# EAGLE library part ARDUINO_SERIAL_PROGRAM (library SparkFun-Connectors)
FTDI connector footprints
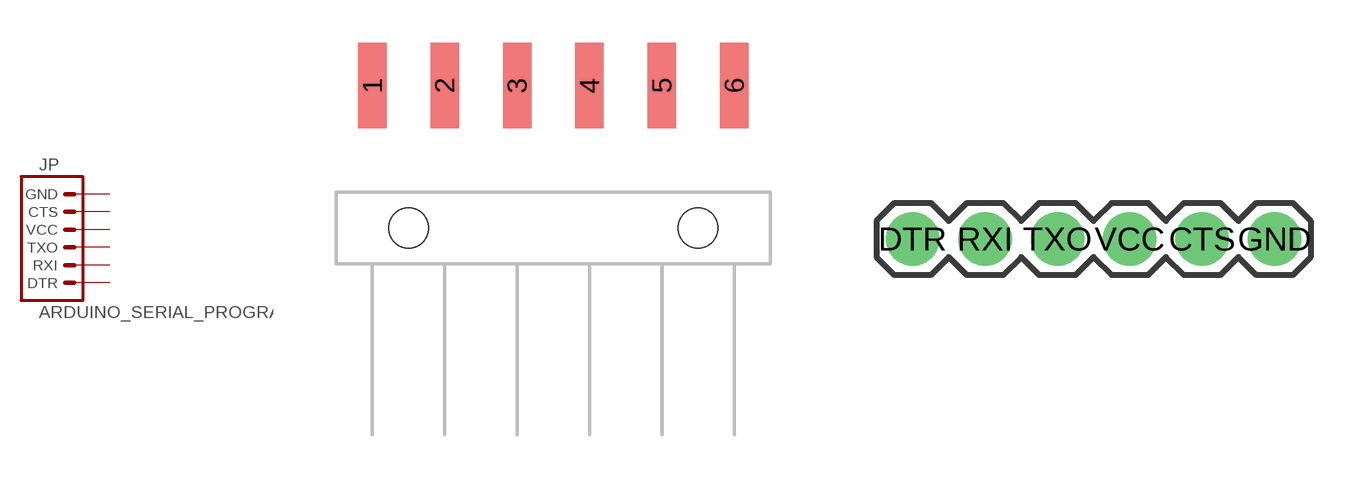
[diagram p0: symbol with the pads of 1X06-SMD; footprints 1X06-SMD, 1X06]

Designator prefix JP

## ARDUINO_SERIAL_PROGRAMSMD  [1X06-SMD]
1  DTR  pas
2  RXI  pas
3  TXO  pas
4  VCC  pas
5  CTS  pas
6  GND  pas

## ARDUINO_SERIAL_PROGRAMPTH  [1X06]
CTS  CTS  pas
DTR  DTR  pas
GND  GND  pas
RXI  RXI  pas
TXO  TXO  pas
VCC  VCC  pas

## ARDUINO_SERIAL_PROGRAMRA_LOCK  [MOLEX-1X6-RA_LOCK]
1  GND  pas
2  CTS  pas
3  VCC  pas
4  TXO  pas
5  RXI  pas
6  DTR  pas

## ARDUINO_SERIAL_PROGRAMLONGPADS  [1X06_LONGPADS]
Pads as for 1X06-SMD

## ARDUINO_SERIAL_PROGRAMLOCK  [1X06_LOCK]
Pads as for 1X06-SMD

## ARDUINO_SERIAL_PROGRAMPTH-KIT  [1X06-KIT]
Pads as for 1X06-SMD

## Footprint 1X06-SMD (pad centres in mm)
smd 1 x 3: 1 -6.35,5; 2 -3.81,5; 3 -1.27,5; 4 1.27,5; 5 3.81,5; 6 6.35,5
hole 1.4 at -5.08,0
hole 1.4 at 5.08,0

## Footprint 1X06 (pad centres in mm)
drill 1.016 pad 1.88: CTS 10.16,0; DTR 0,0; GND 12.7,0; RXI 2.54,0; TXO 5.08,0; VCC 7.62,0

## Footprint MOLEX-1X6-RA_LOCK (pad centres in mm)
drill 1.016 pad 1.88 square: 1 0,0.127
drill 1.016 pad 1.88: 2 2.54,-0.127; 3 5.08,0.127; 4 7.62,-0.127; 5 10.16,0.127; 6 12.7,-0.127

## Footprint 1X06_LONGPADS (pad centres in mm)
drill 1.118 pad 1.88 long: 1 0,0; 2 2.54,0; 3 5.08,0; 4 7.62,0; 5 10.16,0; 6 12.7,0

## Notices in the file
Licensing: Creative Commons ShareAlike 4.0 International - https://creativecommons.org/licenses/by-sa/4.0
